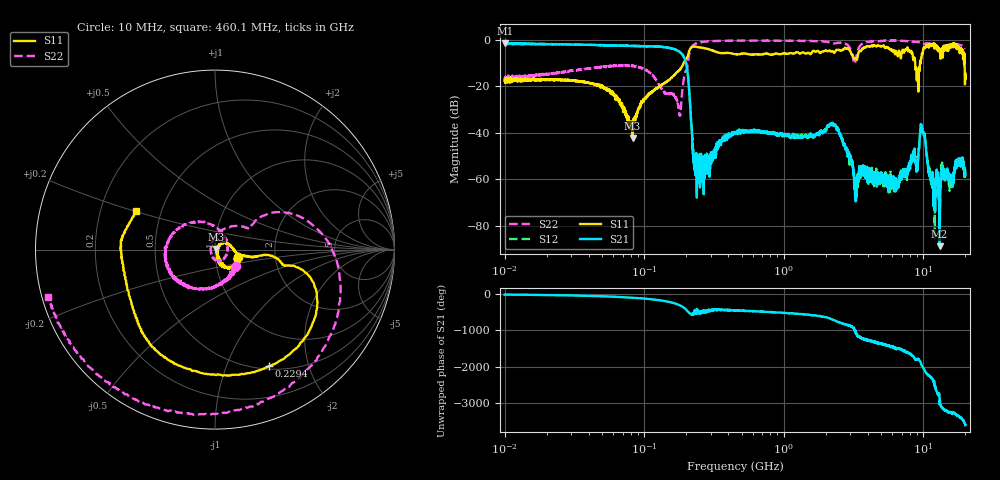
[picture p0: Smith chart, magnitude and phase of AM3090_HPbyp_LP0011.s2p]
# Hz S DB R 50
!freq MagS11 AngS11 MagS21 AngS21 MagS12 AngS12 MagS22 AngS22
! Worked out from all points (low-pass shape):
!   3201 points, 10 MHz to 20 GHz, reference 50 ohm
!   highest |S21| = -1.38 dB at 10.05 MHz (marker M1); lowest = -88.7 dB at 13.07 GHz (marker M2)
!   |S21| within 3 dB of the highest: start of sweep to 170.5 MHz
!   lowest |S11| = -42.2 dB at 82.62 MHz (marker M3), VSWR 1.02, Z = 50.7 + j0.308 ohm
!   |S11| at or under -10 dB: start of sweep to 191.5 MHz; 8.728 GHz to 9.455 GHz (727 MHz wide, 8 % of centre); 19.73 GHz to end of sweep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
!   |S22| runs from -32.5 to -0.2 dB; largest |S21 - S12| = 0.036
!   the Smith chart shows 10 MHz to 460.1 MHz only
!   S11 on the Smith chart (normalised r, x): 10 MHz: 1.29, -0.11; 229.4 MHz: 0.54, -1.43; 460.1 MHz: 0.36, +0.20
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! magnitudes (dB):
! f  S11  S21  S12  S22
! 10 MHz  -17.5  -1.7  -1.6  -16.6
! 10.05 MHz  -16.9  -1.4  -1.7  -17.5
! 35.55 MHz  -18.0  -2.1  -2.0  -12.7
! 82.62 MHz  -42.2  -2.6  -2.5  -11.2
! 126.1 MHz  -20.4  -2.9  -2.9  -18.5
! 177.9 MHz  -13.0  -5.0  -4.9  -31.2
! 195.7 MHz  -8.9  -8.4  -8.3  -14.3
! 229.4 MHz  -2.9  -53.1  -51.1  -1.9
! 447.2 MHz  -6.1  -40.1  -40.2  -0.3
! 460.1 MHz  -6.2  -40.0  -39.8  -0.3
! 1.59 GHz  -5.3  -41.5  -40.8  -0.4
! 2.292 GHz  -5.5  -36.7  -36.3  -1.5
! 3.281 GHz  -7.8  -64.4  -67.5  -8.4
! 3.634 GHz  -3.8  -56.4  -55.2  -1.7
! 5.639 GHz  -3.6  -65.5  -60.7  -0.3
! 7.92 GHz  -4.7  -53.1  -54.2  -0.5
! 8.982 GHz  -17.5  -55.7  -56.1  -0.9
! 9.831 GHz  -6.2  -38.8  -38.5  -1.2
! 11.66 GHz  -2.4  -60.0  -63.9  -2.3
! 13.07 GHz  -4.2  -88.7  -69.0  -3.9
! 17.14 GHz  -2.3  -55.3  -54.2  -1.8
! 20 GHz  -14.4  -58.2  -55.5  -3.6
